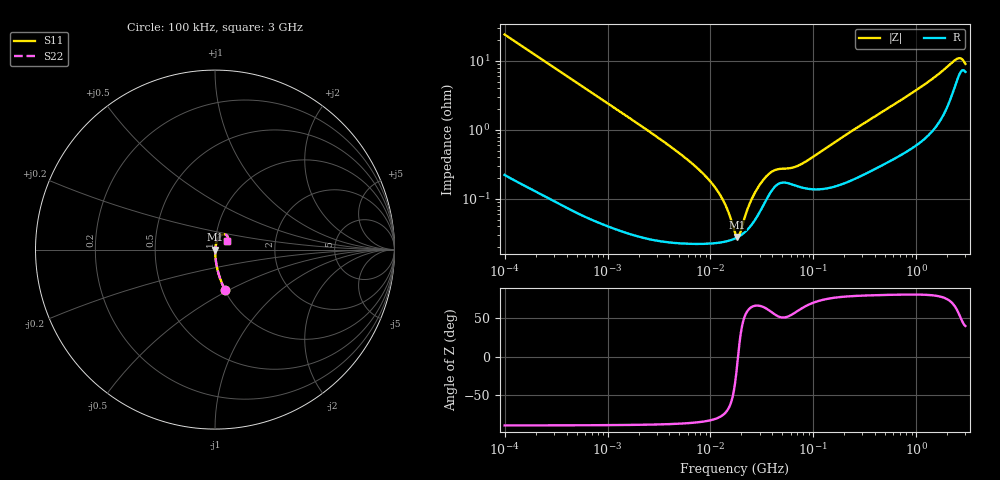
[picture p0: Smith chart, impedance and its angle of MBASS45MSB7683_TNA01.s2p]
! MBASS45MSB7683_TNA01  S-PARAMETER MODEL  ( Standard Model )
! Model Generated by TAIYO YUDEN Corporation (http://www.ty-top.com)
! Version 1.0
! TAIYO YUDEN Control No. 220601
! Copyright(c) 2013 TAIYO YUDEN CO.,LTD. All Rights Reserved.
! Product Description (link to TY-COMPAS)
! https://ds.yuden.co.jp/TYCOMPAS/or/detail?pn=MBASS45MSB7683KTNA01&u=M
! Products Name : Multilayer Ceramic Capacitors
! Characteristics :
!  Capacitance : 0.068 [uF] , Rated Voltage : 630 [V] , TCC : X7R
!  Case Size : 4.5 x 3.2 / 0.177 x 0.126 [mm/inch] , Thickness : 2.5 / 0.098 [mm/inch]
!  (Conditions: Temperature = 25 [degC] , DC Bias Voltage = 0 [V])
! External Node Assignments :
!  1  o---| |---o  2
! GND o---------o GND
! Frequency Range : 100kHz  -  3GHz  [ 401 STEP ]
# MHZ S RI R 50
! Freq[MHz].  S11 Real  S11 Imag  S21 Real  S21 Imag  S12 Real  S12 Imag  S22 Real  S22 Imag
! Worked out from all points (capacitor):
!   401 points, 100 kHz to 3 GHz, reference 50 ohm
!   read as one part in series: C = 65.9 nF near 105.3 kHz
!   lowest |Z| = 28.2 mohm at 18.24 MHz (marker M1)
!   series resonance near 18.53 MHz, so ESL is about 1.1 nH
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0.1  0.0568 -0.2268  0.9432 0.2268  0.9432 0.2268  0.0568 -0.2268
0.222319  0.0129 -0.1073  0.9871 0.1073  0.9871 0.1073  0.0129 -0.1073
0.562235  0.00245 -0.0431  0.9976 0.0431  0.9976 0.0431  0.00245 -0.0431
3.161081  0.000303 -0.00755  0.9997 0.00755  0.9997 0.00755  0.000303 -0.00755
6.504802  0.000235 -0.00334  0.9998 0.00334  0.9998 0.00334  0.000235 -0.00334
10.34438  0.00023 -0.00167  0.9998 0.00167  0.9998 0.00167  0.00023 -0.00167
13.7349  0.000241 -0.000832  0.9998 0.000832  0.9998 0.000832  0.000241 -0.000832
17.7727  0.000273 -0.000116  0.9997 0.000116  0.9997 0.000116  0.000273 -0.000116
18.2367  0.000278 -4.41e-05  0.9997 4.41e-05  0.9997 4.41e-05  0.000278 -4.41e-05
19.70265  0.000298 0.000174  0.9997 -0.000174  0.9997 -0.000174  0.000298 0.000174
22.41241  0.000349 0.000548  0.9997 -0.000548  0.9997 -0.000548  0.000349 0.000548
25.49486  0.000437 0.000941  0.9996 -0.000941  0.9996 -0.000941  0.000437 0.000941
29.75839  0.000629 0.00143  0.9994 -0.00143  0.9994 -0.00143  0.000629 0.00143
34.73492  0.000964 0.00187  0.999 -0.00187  0.999 -0.00187  0.000964 0.00187
41.60216  0.00147 0.00213  0.9985 -0.00213  0.9985 -0.00213  0.00147 0.00213
66.15861  0.00158 0.00244  0.9984 -0.00244  0.9984 -0.00244  0.00158 0.00244
97.38194  0.0014 0.00373  0.9986 -0.00373  0.9986 -0.00373  0.0014 0.00373
547.5153  0.00391 0.0207  0.9961 -0.0207  0.9961 -0.0207  0.00391 0.0207
1249.01  0.00985 0.0459  0.9901 -0.0459  0.9901 -0.0459  0.00985 0.0459
2378.954  0.0489 0.0849  0.9511 -0.0849  0.9511 -0.0849  0.0489 0.0849
2637.286  0.0672 0.0773  0.9328 -0.0773  0.9328 -0.0773  0.0672 0.0773
3000  0.0675 0.0506  0.9325 -0.0506  0.9325 -0.0506  0.0675 0.0506
